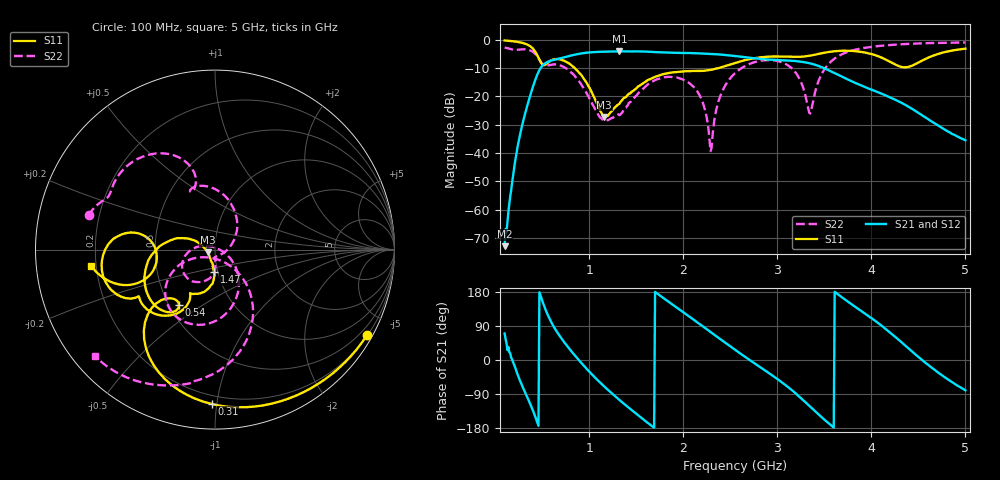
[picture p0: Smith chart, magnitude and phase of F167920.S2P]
!  2-Port S-parameters saved by WinCal
! VAR MeasName=S-Parameters (CALIBRATED_DATA) read from VNA (N5242A)
! VAR MeasDate=2016-11-22 9:53:28
! VAR NAME=F167920
! VAR FILENAME=F167920.S2P
! VAR DATE=2016-11-22 9:53:28
! VAR PHYS_PORTS=1,2
# Hz S DB R 50
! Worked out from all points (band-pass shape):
!   491 points, 100 MHz to 5 GHz, reference 50 ohm
!   highest |S21| = -4.08 dB at 1.32 GHz (marker M1); lowest = -73.0 dB at 100 MHz (marker M2)
!   |S21| within 3 dB of the highest: 628.8 MHz to 2.943 GHz (2.314 GHz wide, 130 % of centre)
!   lowest |S11| = -27.3 dB at 1.16 GHz (marker M3), VSWR 1.09, Z = 46.1 - j1.35 ohm
!   |S11| at or under -10 dB: 845.7 MHz to 2.377 GHz (1.532 GHz wide, 95 % of centre)
!   |S22| runs from -39.4 to -1.0 dB; largest |S21 - S12| = 0.0017
!   S11 on the Smith chart (normalised r, x): 100 MHz: 0.22, -3.82; 310 MHz: 0.15, -0.97; 540 MHz: 0.56, -0.40; 1.47 GHz: 0.96, -0.25; 5 GHz: 0.18, -0.06
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1e8  -0.25 -29.3  -72.95 70.0  -70.01 70.2  -2.74 164.7
2.2e8  -0.67 -63.8  -41.32 -25.6  -41.29 -25.5  -3.57 152.3
3.1e8  -1.31 -91.2  -27.12 -81.2  -27.14 -81.1  -3.37 139.6
4.2e8  -3.93 -128.4  -14.75 -145.4  -14.74 -145.3  -4.81 113.7
5.4e8  -8.66 -122.9  -8.11 130.0  -8.10 130.0  -9.15 112.0
6.9e8  -6.96 -147.6  -6.58 61.9  -6.57 61.9  -9.04 96.2
9.2e8  -12.63 165.1  -4.80 -8.8  -4.80 -8.8  -16.08 39.7
1.16e9  -27.29 -160.2  -4.20 -70.1  -4.19 -70.1  -28.59 -63.2
1.32e9  -22.65 -102.4  -4.08 -105.0  -4.07 -105.0  -26.63 -95.8
1.47e9  -17.97 -92.5  -4.13 -135.8  -4.12 -135.8  -20.79 -89.0
1.74e9  -12.64 -102.3  -4.41 172.3  -4.41 172.3  -13.77 -117.9
2.13e9  -11.04 -119.7  -4.76 102.8  -4.75 102.7  -17.36 -178.9
2.22e9  -10.96 -119.3  -4.88 86.6  -4.87 86.6  -23.49 161.8
2.29e9  -10.65 -118.0  -4.98 73.9  -4.98 73.8  -39.38 86.7
2.39e9  -9.88 -116.6  -5.21 55.6  -5.20 55.6  -20.18 -29.8
2.55e9  -8.19 -118.8  -5.75 26.9  -5.74 26.9  -11.82 -59.3
3.06e9  -5.93 -144.8  -7.27 -61.0  -7.26 -61.1  -8.12 -133.9
3.37e9  -5.49 -149.3  -8.54 -127.8  -8.51 -127.9  -23.43 -63.8
3.46e9  -4.86 -152.0  -9.54 -148.4  -9.51 -148.6  -12.87 -46.2
3.6e9  -4.09 -159.9  -11.61 -178.1  -11.60 -178.3  -6.87 -62.8
4.19e9  -7.64 168.4  -20.22 74.4  -20.22 74.3  -1.88 -109.9
5e9  -3.15 -172.5  -35.54 -80.2  -35.53 -79.9  -0.97 -138.5
